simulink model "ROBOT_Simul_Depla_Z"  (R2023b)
settings: Solver=ode15s  StartTime=0.0  StopTime=0.2  RelTol=1e-3  EnableMultiTasking=on
undefined symbols (not defined in the file): BATI1_Défaut_sldprt, BATI2_Défaut_sldprt, BATI3_Défaut_sldprt, deg, kg, m, mm, N, rad, s, STL, X, Y, Z
libraries: sm_lib x139, fl_lib x42, nesl_utility x19, slpidlib x3
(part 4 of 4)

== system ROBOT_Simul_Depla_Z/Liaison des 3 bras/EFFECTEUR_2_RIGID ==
  ReferenceFrame : sm_lib/Frames and Transforms/Reference Frame
  Solid : sm_lib/Body Elements/File Solid  ExtGeomFileName=\STL\EFFECTEUR_Défaut_sldprt.STL  UnitType=Custom  ExtGeomFileUnits=mm  StepReaderType=HEX  ExportConvexHullGeometry=off  InertiaType=Custom  Mass=0.013453568991832839  MassUnits=kg  CenterOfMass=[-17.212650388480686 -9.9626588451280398 5.5774208666899616]  CenterOfMassUnits=mm  MomentsOfInertia=[1.2849612996466211 1.3154199043910564 2.2338709867359823]  MomentsOfInertiaUnits=kg*mm^2  ProductsOfInertia=[0.035925388048610812 0.056750034506765974 -0.058662844210309435]  ProductsOfInertiaUnits=kg*mm^2  BasedOnType=Density  Density=1000  DensityUnits=kg/(m^3)  DoExposeReferenceFrame=on  SerializedFrames=<Frames/>  GraphicType=FromGeometry  MarkerShape=Sphere  MarkerSize=10  MarkerSizeUnits=m  GraphicVisPropType=SimpleVisualProperties  GraphicDiffuseColor=[0.792156862745098 0.81960784313725488 0.93333333333333335]  GraphicSpecularColor=[0.5 0.5 0.5 1.0]  GraphicAmbientColor=[0.15 0.15 0.15 1.0]  GraphicEmissiveColor=[0.0 0.0 0.0 1.0]  GraphicShininess=75  GraphicOpacity=1
  F : PMIOPort  Side=Left
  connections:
  Solid/RConn1 -- ReferenceFrame/RConn1 -- F/RConn1

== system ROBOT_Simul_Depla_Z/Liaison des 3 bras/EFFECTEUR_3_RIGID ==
  ReferenceFrame : sm_lib/Frames and Transforms/Reference Frame
  Solid : sm_lib/Body Elements/File Solid  ExtGeomFileName=\STL\EFFECTEUR_Défaut_sldprt.STL  UnitType=Custom  ExtGeomFileUnits=mm  StepReaderType=HEX  ExportConvexHullGeometry=off  InertiaType=Custom  Mass=0.013453568991832839  MassUnits=kg  CenterOfMass=[-17.212650388480686 -9.9626588451280398 5.5774208666899616]  CenterOfMassUnits=mm  MomentsOfInertia=[1.2849612996466211 1.3154199043910564 2.2338709867359823]  MomentsOfInertiaUnits=kg*mm^2  ProductsOfInertia=[0.035925388048610812 0.056750034506765974 -0.058662844210309435]  ProductsOfInertiaUnits=kg*mm^2  BasedOnType=Density  Density=1000  DensityUnits=kg/(m^3)  DoExposeReferenceFrame=on  SerializedFrames=<Frames/>  GraphicType=FromGeometry  MarkerShape=Sphere  MarkerSize=10  MarkerSizeUnits=m  GraphicVisPropType=SimpleVisualProperties  GraphicDiffuseColor=[0.792156862745098 0.81960784313725488 0.93333333333333335]  GraphicSpecularColor=[0.5 0.5 0.5 1.0]  GraphicAmbientColor=[0.15 0.15 0.15 1.0]  GraphicEmissiveColor=[0.0 0.0 0.0 1.0]  GraphicShininess=75  GraphicOpacity=1
  F : PMIOPort  Side=Left
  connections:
  Solid/RConn1 -- ReferenceFrame/RConn1 -- F/RConn1

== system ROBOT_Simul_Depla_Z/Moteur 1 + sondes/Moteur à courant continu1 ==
  note: Kv = 1.18e-1
  Frottement : fl_lib/Mechanical/Rotational Elements/Rotational Friction  brkwy_trq=2.43e-3 N*m  brkwy_vel=0.030296 rad/s  Col_trq=2.43e-3 N*m  visc_coef=2e-6 N*m/(rad/s)  w_specify=off  w_priority=None  w=0 rad/s  w_nominal_specify=off  w_nominal_unit=rad/s  w_nominal_value=1  t_specify=off  t_priority=None  t=0 N*m  t_nominal_specify=off  t_nominal_unit=N*m  t_nominal_value=1
  Inductance induit 35mH : fl_lib/Electrical/Electrical Elements/Inductor  l=35 mH  r=0 Ohm  g=1e-09 1/Ohm  i_specify=off  i_priority=None  i=0 A  i_nominal_specify=off  i_nominal_unit=A  i_nominal_value=1  v_specify=off  v_priority=None  v=0 V  v_nominal_specify=off  v_nominal_unit=V  v_nominal_value=1  i_L_specify=on  i_L_priority=High  i_L=0 A  i_L_nominal_specify=off  i_L_nominal_unit=A  i_L_nominal_value=1
  Inertie Je 10e-6 : fl_lib/Mechanical/Rotational Elements/Inertia  inertia=10.5e-6 kg*m^2  num_ports=foundation.enum.numPorts2.one  w_specify=on  w_priority=High  w=0 rad/s  w_nominal_specify=off  w_nominal_unit=rad/s  w_nominal_value=1  t_specify=off  t_priority=None  t=0 N*m  t_nominal_specify=off  t_nominal_unit=N*m  t_nominal_value=1
  Moteur parfait : fl_lib/Electrical/Electrical Elements/Rotational Electromechanical Converter  K=1.18e-1 V/(rad/s)  i_specify=off  i_priority=None  i=0 A  i_nominal_specify=off  i_nominal_unit=A  i_nominal_value=1  v_specify=off  v_priority=None  v=0 V  v_nominal_specify=off  v_nominal_unit=V  v_nominal_value=1  t_specify=off  t_priority=None  t=0 N*m  t_nominal_specify=off  t_nominal_unit=N*m  t_nominal_value=1  w_specify=off  w_priority=None  w=0 rad/s  w_nominal_specify=off  w_nominal_unit=rad/s  w_nominal_value=1
  Rinduit 38 Ohms : fl_lib/Electrical/Electrical Elements/Resistor  Tag=Factory Generic  R=38 Ohm  i_specify=off  i_priority=None  i=0 A  i_nominal_specify=off  i_nominal_unit=A  i_nominal_value=1  v_specify=off  v_priority=None  v=0 V  v_nominal_specify=off  v_nominal_unit=V  v_nominal_value=1
  V+ : PMIOPort  Side=Left
  R : PMIOPort  Port=2  Side=Right
  C : PMIOPort  Port=3  Side=Right
  V- : PMIOPort  Port=4  Side=Left
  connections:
  C/RConn1 -- Moteur parfait/RConn2 -- Frottement/RConn1
  R/RConn1 -- Inertie Je 10e-6/LConn1 -- Moteur parfait/LConn2 -- Frottement/LConn1
  Inductance induit 35mH/LConn1 -- Rinduit 38 Ohms/RConn1
  Rinduit 38 Ohms/LConn1 -- V+/RConn1
  V-/RConn1 -- Moteur parfait/RConn1
  Moteur parfait/LConn1 -- Inductance induit 35mH/RConn1

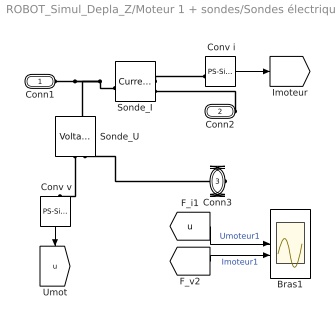
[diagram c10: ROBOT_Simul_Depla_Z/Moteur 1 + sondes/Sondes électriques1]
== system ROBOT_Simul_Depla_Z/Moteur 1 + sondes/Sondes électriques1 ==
  " Conv i" : nesl_utility/PS-Simulink Converter  PhysicalDomain=network_engine_domain  SubClassName=ps_output  LeftPortType=input  RightPortType=output  PseudoPeriodic=off  Frequencies=[]  VectorFormat=1-D array  Unit=1  AffineConversion=off
  " Conv v" : nesl_utility/PS-Simulink Converter  PhysicalDomain=network_engine_domain  SubClassName=ps_output  LeftPortType=input  RightPortType=output  PseudoPeriodic=off  Frequencies=[]  VectorFormat=1-D array  Unit=1  AffineConversion=off
  Bras1 : Scope  NumInputPorts=2
  Sonde_I : fl_lib/Electrical/Electrical Sensors/Current Sensor
  Sonde_U : fl_lib/Electrical/Electrical Sensors/Voltage Sensor
  Conn1 : PMIOPort  Side=Left
  Conn2 : PMIOPort  Port=2  Side=Right
  Conn3 : PMIOPort  Port=3  Side=Right
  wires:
  [i] -> Bras1/2  "Imoteur1"
  [u] -> Bras1/1  "Umoteur1"
  " Conv i"/1 -> [i]
  " Conv v"/1 -> [u]
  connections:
  Conn3/RConn1 -- Sonde_U/RConn2
  Conn2/RConn1 -- Sonde_I/RConn2
  Sonde_I/LConn1 -- Sonde_U/LConn1 -- Conn1/RConn1
  Sonde_U/RConn1 -- " Conv v"/LConn1
  Sonde_I/RConn1 -- " Conv i"/LConn1

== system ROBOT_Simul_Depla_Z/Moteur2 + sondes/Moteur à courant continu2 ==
  note: Kv = 1.18e-1
  Frottement : fl_lib/Mechanical/Rotational Elements/Rotational Friction  brkwy_trq=2.43e-3 N*m  brkwy_vel=0.030296 rad/s  Col_trq=2.43e-3 N*m  visc_coef=2e-6 N*m/(rad/s)  w_specify=off  w_priority=None  w=0 rad/s  w_nominal_specify=off  w_nominal_unit=rad/s  w_nominal_value=1  t_specify=off  t_priority=None  t=0 N*m  t_nominal_specify=off  t_nominal_unit=N*m  t_nominal_value=1
  Inductance induit 35mH : fl_lib/Electrical/Electrical Elements/Inductor  l=35 mH  r=0 Ohm  g=1e-09 1/Ohm  i_specify=off  i_priority=None  i=0 A  i_nominal_specify=off  i_nominal_unit=A  i_nominal_value=1  v_specify=off  v_priority=None  v=0 V  v_nominal_specify=off  v_nominal_unit=V  v_nominal_value=1  i_L_specify=on  i_L_priority=High  i_L=0 A  i_L_nominal_specify=off  i_L_nominal_unit=A  i_L_nominal_value=1
  Inertie Je 10e-6 : fl_lib/Mechanical/Rotational Elements/Inertia  inertia=10.5e-6 kg*m^2  num_ports=foundation.enum.numPorts2.one  w_specify=on  w_priority=High  w=0 rad/s  w_nominal_specify=off  w_nominal_unit=rad/s  w_nominal_value=1  t_specify=off  t_priority=None  t=0 N*m  t_nominal_specify=off  t_nominal_unit=N*m  t_nominal_value=1
  Moteur parfait : fl_lib/Electrical/Electrical Elements/Rotational Electromechanical Converter  K=1.18e-1 V/(rad/s)  i_specify=off  i_priority=None  i=0 A  i_nominal_specify=off  i_nominal_unit=A  i_nominal_value=1  v_specify=off  v_priority=None  v=0 V  v_nominal_specify=off  v_nominal_unit=V  v_nominal_value=1  t_specify=off  t_priority=None  t=0 N*m  t_nominal_specify=off  t_nominal_unit=N*m  t_nominal_value=1  w_specify=off  w_priority=None  w=0 rad/s  w_nominal_specify=off  w_nominal_unit=rad/s  w_nominal_value=1
  Rinduit 38 Ohms : fl_lib/Electrical/Electrical Elements/Resistor  Tag=Factory Generic  R=38 Ohm  i_specify=off  i_priority=None  i=0 A  i_nominal_specify=off  i_nominal_unit=A  i_nominal_value=1  v_specify=off  v_priority=None  v=0 V  v_nominal_specify=off  v_nominal_unit=V  v_nominal_value=1
  V+ : PMIOPort  Side=Left
  R : PMIOPort  Port=2  Side=Right
  C : PMIOPort  Port=3  Side=Right
  V- : PMIOPort  Port=4  Side=Left
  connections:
  Moteur parfait/LConn1 -- Inductance induit 35mH/RConn1
  V-/RConn1 -- Moteur parfait/RConn1
  Rinduit 38 Ohms/LConn1 -- V+/RConn1
  Inductance induit 35mH/LConn1 -- Rinduit 38 Ohms/RConn1
  Frottement/LConn1 -- Moteur parfait/LConn2 -- Inertie Je 10e-6/LConn1 -- R/RConn1
  Frottement/RConn1 -- Moteur parfait/RConn2 -- C/RConn1

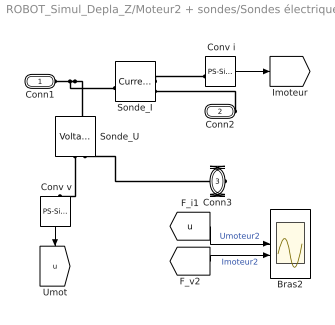
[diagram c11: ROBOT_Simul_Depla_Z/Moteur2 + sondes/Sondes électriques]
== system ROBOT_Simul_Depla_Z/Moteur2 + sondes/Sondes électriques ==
  " Conv i" : nesl_utility/PS-Simulink Converter  PhysicalDomain=network_engine_domain  SubClassName=ps_output  LeftPortType=input  RightPortType=output  PseudoPeriodic=off  Frequencies=[]  VectorFormat=1-D array  Unit=1  AffineConversion=off
  " Conv v" : nesl_utility/PS-Simulink Converter  PhysicalDomain=network_engine_domain  SubClassName=ps_output  LeftPortType=input  RightPortType=output  PseudoPeriodic=off  Frequencies=[]  VectorFormat=1-D array  Unit=1  AffineConversion=off
  Bras2 : Scope  NumInputPorts=2
  Sonde_I : fl_lib/Electrical/Electrical Sensors/Current Sensor
  Sonde_U : fl_lib/Electrical/Electrical Sensors/Voltage Sensor
  Conn1 : PMIOPort  Side=Left
  Conn2 : PMIOPort  Port=2  Side=Right
  Conn3 : PMIOPort  Port=3  Side=Right
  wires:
  " Conv v"/1 -> [u]
  " Conv i"/1 -> [i]
  [u] -> Bras2/1  "Umoteur2"
  [i] -> Bras2/2  "Imoteur2"
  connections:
  Sonde_I/RConn1 -- " Conv i"/LConn1
  Sonde_U/RConn1 -- " Conv v"/LConn1
  Conn1/RConn1 -- Sonde_U/LConn1 -- Sonde_I/LConn1
  Conn2/RConn1 -- Sonde_I/RConn2
  Conn3/RConn1 -- Sonde_U/RConn2

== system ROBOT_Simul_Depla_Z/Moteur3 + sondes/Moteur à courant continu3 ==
  note: Kv = 1.18e-1
  Frottement : fl_lib/Mechanical/Rotational Elements/Rotational Friction  brkwy_trq=2.43e-3 N*m  brkwy_vel=0.030296 rad/s  Col_trq=2.43e-3 N*m  visc_coef=2e-6 N*m/(rad/s)  w_specify=off  w_priority=None  w=0 rad/s  w_nominal_specify=off  w_nominal_unit=rad/s  w_nominal_value=1  t_specify=off  t_priority=None  t=0 N*m  t_nominal_specify=off  t_nominal_unit=N*m  t_nominal_value=1
  Inductance induit 35mH : fl_lib/Electrical/Electrical Elements/Inductor  l=35 mH  r=0 Ohm  g=1e-09 1/Ohm  i_specify=off  i_priority=None  i=0 A  i_nominal_specify=off  i_nominal_unit=A  i_nominal_value=1  v_specify=off  v_priority=None  v=0 V  v_nominal_specify=off  v_nominal_unit=V  v_nominal_value=1  i_L_specify=on  i_L_priority=High  i_L=0 A  i_L_nominal_specify=off  i_L_nominal_unit=A  i_L_nominal_value=1
  Inertie Je 10e-6 : fl_lib/Mechanical/Rotational Elements/Inertia  inertia=10.5e-6 kg*m^2  num_ports=foundation.enum.numPorts2.one  w_specify=on  w_priority=High  w=0 rad/s  w_nominal_specify=off  w_nominal_unit=rad/s  w_nominal_value=1  t_specify=off  t_priority=None  t=0 N*m  t_nominal_specify=off  t_nominal_unit=N*m  t_nominal_value=1
  Moteur parfait : fl_lib/Electrical/Electrical Elements/Rotational Electromechanical Converter  K=1.18e-1 V/(rad/s)  i_specify=off  i_priority=None  i=0 A  i_nominal_specify=off  i_nominal_unit=A  i_nominal_value=1  v_specify=off  v_priority=None  v=0 V  v_nominal_specify=off  v_nominal_unit=V  v_nominal_value=1  t_specify=off  t_priority=None  t=0 N*m  t_nominal_specify=off  t_nominal_unit=N*m  t_nominal_value=1  w_specify=off  w_priority=None  w=0 rad/s  w_nominal_specify=off  w_nominal_unit=rad/s  w_nominal_value=1
  Rinduit 38 Ohms : fl_lib/Electrical/Electrical Elements/Resistor  Tag=Factory Generic  R=38 Ohm  i_specify=off  i_priority=None  i=0 A  i_nominal_specify=off  i_nominal_unit=A  i_nominal_value=1  v_specify=off  v_priority=None  v=0 V  v_nominal_specify=off  v_nominal_unit=V  v_nominal_value=1
  V+ : PMIOPort  Side=Left
  R : PMIOPort  Port=2  Side=Right
  C : PMIOPort  Port=3  Side=Right
  V- : PMIOPort  Port=4  Side=Left
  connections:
  Moteur parfait/LConn1 -- Inductance induit 35mH/RConn1
  V-/RConn1 -- Moteur parfait/RConn1
  Rinduit 38 Ohms/LConn1 -- V+/RConn1
  Inductance induit 35mH/LConn1 -- Rinduit 38 Ohms/RConn1
  Frottement/LConn1 -- Moteur parfait/LConn2 -- Inertie Je 10e-6/LConn1 -- R/RConn1
  Frottement/RConn1 -- Moteur parfait/RConn2 -- C/RConn1

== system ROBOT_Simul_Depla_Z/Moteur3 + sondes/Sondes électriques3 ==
  " Conv i" : nesl_utility/PS-Simulink Converter  PhysicalDomain=network_engine_domain  SubClassName=ps_output  LeftPortType=input  RightPortType=output  PseudoPeriodic=off  Frequencies=[]  VectorFormat=1-D array  Unit=1  AffineConversion=off
  " Conv v" : nesl_utility/PS-Simulink Converter  PhysicalDomain=network_engine_domain  SubClassName=ps_output  LeftPortType=input  RightPortType=output  PseudoPeriodic=off  Frequencies=[]  VectorFormat=1-D array  Unit=1  AffineConversion=off
  Bras3 : Scope  NumInputPorts=2
  Sonde_I : fl_lib/Electrical/Electrical Sensors/Current Sensor
  Sonde_U : fl_lib/Electrical/Electrical Sensors/Voltage Sensor
  Conn1 : PMIOPort  Side=Left
  Conn2 : PMIOPort  Port=2  Side=Right
  Conn3 : PMIOPort  Port=3  Side=Right
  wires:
  " Conv v"/1 -> [u]
  " Conv i"/1 -> [i]
  [u] -> Bras3/1  "Umoteur3"
  [i] -> Bras3/2  "Imoteur3"
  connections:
  Sonde_I/RConn1 -- " Conv i"/LConn1
  Sonde_U/RConn1 -- " Conv v"/LConn1
  Conn1/RConn1 -- Sonde_U/LConn1 -- Sonde_I/LConn1
  Conn2/RConn1 -- Sonde_I/RConn2
  Conn3/RConn1 -- Sonde_U/RConn2

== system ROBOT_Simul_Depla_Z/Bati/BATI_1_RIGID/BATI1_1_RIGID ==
  ReferenceFrame : sm_lib/Frames and Transforms/Reference Frame
  Solid : sm_lib/Body Elements/File Solid  ExtGeomFileName=\STL\BATI1_Défaut_sldprt.STL  UnitType=Custom  ExtGeomFileUnits=mm  StepReaderType=HEX  ExportConvexHullGeometry=off  InertiaType=Custom  Mass=0.033663687372977959  MassUnits=kg  CenterOfMass=[20.336401330469712 25.63961437498785 5.3457144153831457]  CenterOfMassUnits=mm  MomentsOfInertia=[6.704545070550517 14.392527306394198 20.235421331927157]  MomentsOfInertiaUnits=kg*mm^2  ProductsOfInertia=[-0.10543470284856278 -0.074747369019470072 1.7068027580925555]  ProductsOfInertiaUnits=kg*mm^2  BasedOnType=Density  Density=1000  DensityUnits=kg/(m^3)  DoExposeReferenceFrame=on  SerializedFrames=<Frames/>  GraphicType=FromGeometry  MarkerShape=Sphere  MarkerSize=10  MarkerSizeUnits=m  GraphicVisPropType=SimpleVisualProperties  GraphicDiffuseColor=[0.75294117647058822 1 1]  GraphicSpecularColor=[0.5 0.5 0.5 1.0]  GraphicAmbientColor=[0.15 0.15 0.15 1.0]  GraphicEmissiveColor=[0.0 0.0 0.0 1.0]  GraphicShininess=75  GraphicOpacity=1
  F : PMIOPort  Side=Left
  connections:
  Solid/RConn1 -- ReferenceFrame/RConn1 -- F/RConn1

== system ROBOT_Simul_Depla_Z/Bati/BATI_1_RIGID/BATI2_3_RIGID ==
  ReferenceFrame : sm_lib/Frames and Transforms/Reference Frame
  Solid : sm_lib/Body Elements/File Solid  ExtGeomFileName=\STL\BATI2_Défaut_sldprt.STL  UnitType=Custom  ExtGeomFileUnits=mm  StepReaderType=HEX  ExportConvexHullGeometry=off  InertiaType=Custom  Mass=3.3661932429020234  MassUnits=kg  CenterOfMass=[20.336944533823793 25.639868756108907 5.3454769419575205]  CenterOfMassUnits=mm  MomentsOfInertia=[670.44550783613272 1439.2294811094996 2023.5171686685317]  MomentsOfInertiaUnits=kg*mm^2  ProductsOfInertia=[-10.547370497314642 -7.4830660580031543 170.68937998442982]  ProductsOfInertiaUnits=kg*mm^2  BasedOnType=Density  Density=1000  DensityUnits=kg/(m^3)  DoExposeReferenceFrame=on  SerializedFrames=<Frames/>  GraphicType=FromGeometry  MarkerShape=Sphere  MarkerSize=10  MarkerSizeUnits=m  GraphicVisPropType=SimpleVisualProperties  GraphicDiffuseColor=[0.75294117647058822 1 1]  GraphicSpecularColor=[0.5 0.5 0.5 1.0]  GraphicAmbientColor=[0.15 0.15 0.15 1.0]  GraphicEmissiveColor=[0.0 0.0 0.0 1.0]  GraphicShininess=75  GraphicOpacity=1
  F : PMIOPort  Side=Left
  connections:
  Solid/RConn1 -- ReferenceFrame/RConn1 -- F/RConn1

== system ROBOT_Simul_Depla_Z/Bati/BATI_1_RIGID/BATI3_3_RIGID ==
  ReferenceFrame : sm_lib/Frames and Transforms/Reference Frame
  Solid : sm_lib/Body Elements/File Solid  ExtGeomFileName=\STL\BATI3_Défaut_sldprt.STL  UnitType=Custom  ExtGeomFileUnits=mm  StepReaderType=HEX  ExportConvexHullGeometry=off  InertiaType=Custom  Mass=0.033661997544023686  MassUnits=kg  CenterOfMass=[20.336894016558855 25.639858086732207 5.3454859216357811]  CenterOfMassUnits=mm  MomentsOfInertia=[6.7044612586719987 14.392323903610993 20.235203785272009]  MomentsOfInertiaUnits=kg*mm^2  ProductsOfInertia=[-0.10547223942223864 -0.074822963165538006 1.706885098239038]  ProductsOfInertiaUnits=kg*mm^2  BasedOnType=Density  Density=1000  DensityUnits=kg/(m^3)  DoExposeReferenceFrame=on  SerializedFrames=<Frames/>  GraphicType=FromGeometry  MarkerShape=Sphere  MarkerSize=10  MarkerSizeUnits=m  GraphicVisPropType=SimpleVisualProperties  GraphicDiffuseColor=[0.75294117647058822 1 1]  GraphicSpecularColor=[0.5 0.5 0.5 1.0]  GraphicAmbientColor=[0.15 0.15 0.15 1.0]  GraphicEmissiveColor=[0.0 0.0 0.0 1.0]  GraphicShininess=75  GraphicOpacity=1
  F : PMIOPort  Side=Left
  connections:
  Solid/RConn1 -- ReferenceFrame/RConn1 -- F/RConn1

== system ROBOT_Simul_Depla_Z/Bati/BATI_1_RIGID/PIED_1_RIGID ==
  ReferenceFrame : sm_lib/Frames and Transforms/Reference Frame
  Solid : sm_lib/Body Elements/File Solid  ExtGeomFileName=\STL\PIED_Défaut_sldprt.STL  UnitType=Custom  ExtGeomFileUnits=mm  StepReaderType=HEX  ExportConvexHullGeometry=off  InertiaType=Custom  Mass=0.2400116994364806  MassUnits=kg  CenterOfMass=[-3.023797205330788 -10.775136940876026 -9.5034409989686353]  CenterOfMassUnits=mm  MomentsOfInertia=[1039.4350917464089 990.05262981218959 1785.3677193958695]  MomentsOfInertiaUnits=kg*mm^2  ProductsOfInertia=[91.936760537551947 25.766048207439965 -15.325521737410117]  ProductsOfInertiaUnits=kg*mm^2  BasedOnType=Density  Density=1000  DensityUnits=kg/(m^3)  DoExposeReferenceFrame=on  SerializedFrames=<Frames/>  GraphicType=FromGeometry  MarkerShape=Sphere  MarkerSize=10  MarkerSizeUnits=m  GraphicVisPropType=SimpleVisualProperties  GraphicDiffuseColor=[0.75294117647058822 1 1]  GraphicSpecularColor=[0.5 0.5 0.5 1.0]  GraphicAmbientColor=[0.15 0.15 0.15 1.0]  GraphicEmissiveColor=[0.0 0.0 0.0 1.0]  GraphicShininess=75  GraphicOpacity=1
  F : PMIOPort  Side=Left
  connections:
  Solid/RConn1 -- ReferenceFrame/RConn1 -- F/RConn1

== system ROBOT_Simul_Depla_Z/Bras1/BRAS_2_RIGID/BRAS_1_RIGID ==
  ReferenceFrame : sm_lib/Frames and Transforms/Reference Frame
  Solid : sm_lib/Body Elements/File Solid  ExtGeomFileName=\STL\BRAS_Défaut_sldprt.STL  UnitType=Custom  ExtGeomFileUnits=mm  StepReaderType=HEX  ExportConvexHullGeometry=off  InertiaType=Custom  Mass=0.044838950955509597  MassUnits=kg  CenterOfMass=[-9.0418534412108452e-05 8.4657112225167754 0.00015611796423892563]  CenterOfMassUnits=mm  MomentsOfInertia=[5.1909513043126365 1.33138621334256 4.0048796257842971]  MomentsOfInertiaUnits=kg*mm^2  ProductsOfInertia=[-7.521699658868721e-06 -1.2077060782263442e-05 -1.0591378087356949e-05]  ProductsOfInertiaUnits=kg*mm^2  BasedOnType=Density  Density=1000  DensityUnits=kg/(m^3)  DoExposeReferenceFrame=on  SerializedFrames=<Frames/>  GraphicType=FromGeometry  MarkerShape=Sphere  MarkerSize=10  MarkerSizeUnits=m  GraphicVisPropType=SimpleVisualProperties  GraphicDiffuseColor=[0.69803921568627447 0.69803921568627447 0.69803921568627447]  GraphicSpecularColor=[0.5 0.5 0.5 1.0]  GraphicAmbientColor=[0.15 0.15 0.15 1.0]  GraphicEmissiveColor=[0.0 0.0 0.0 1.0]  GraphicShininess=75  GraphicOpacity=1
  F : PMIOPort  Side=Left
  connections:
  Solid/RConn1 -- ReferenceFrame/RConn1 -- F/RConn1

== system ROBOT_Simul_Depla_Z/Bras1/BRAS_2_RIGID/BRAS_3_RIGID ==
  ReferenceFrame : sm_lib/Frames and Transforms/Reference Frame
  Solid : sm_lib/Body Elements/File Solid  ExtGeomFileName=\STL\BRAS_Défaut_sldprt.STL  UnitType=Custom  ExtGeomFileUnits=mm  StepReaderType=HEX  ExportConvexHullGeometry=off  InertiaType=Custom  Mass=0.044838950955509597  MassUnits=kg  CenterOfMass=[-9.0418534412108452e-05 8.4657112225167754 0.00015611796423892563]  CenterOfMassUnits=mm  MomentsOfInertia=[5.1909513043126365 1.33138621334256 4.0048796257842971]  MomentsOfInertiaUnits=kg*mm^2  ProductsOfInertia=[-7.521699658868721e-06 -1.2077060782263442e-05 -1.0591378087356949e-05]  ProductsOfInertiaUnits=kg*mm^2  BasedOnType=Density  Density=1000  DensityUnits=kg/(m^3)  DoExposeReferenceFrame=on  SerializedFrames=<Frames/>  GraphicType=FromGeometry  MarkerShape=Sphere  MarkerSize=10  MarkerSizeUnits=m  GraphicVisPropType=SimpleVisualProperties  GraphicDiffuseColor=[0.6 0.6 0.6]  GraphicSpecularColor=[0.5 0.5 0.5 1.0]  GraphicAmbientColor=[0.15 0.15 0.15 1.0]  GraphicEmissiveColor=[0.0 0.0 0.0 1.0]  GraphicShininess=75  GraphicOpacity=1
  F : PMIOPort  Side=Left
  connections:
  Solid/RConn1 -- ReferenceFrame/RConn1 -- F/RConn1

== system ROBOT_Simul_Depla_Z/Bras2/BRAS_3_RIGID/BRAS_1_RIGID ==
  ReferenceFrame : sm_lib/Frames and Transforms/Reference Frame
  Solid : sm_lib/Body Elements/File Solid  ExtGeomFileName=\STL\BRAS_Défaut_sldprt.STL  UnitType=Custom  ExtGeomFileUnits=mm  StepReaderType=HEX  ExportConvexHullGeometry=off  InertiaType=Custom  Mass=0.044838950955509597  MassUnits=kg  CenterOfMass=[-9.0418534412108452e-05 8.4657112225167754 0.00015611796423892563]  CenterOfMassUnits=mm  MomentsOfInertia=[5.1909513043126365 1.33138621334256 4.0048796257842971]  MomentsOfInertiaUnits=kg*mm^2  ProductsOfInertia=[-7.521699658868721e-06 -1.2077060782263442e-05 -1.0591378087356949e-05]  ProductsOfInertiaUnits=kg*mm^2  BasedOnType=Density  Density=1000  DensityUnits=kg/(m^3)  DoExposeReferenceFrame=on  SerializedFrames=<Frames/>  GraphicType=FromGeometry  MarkerShape=Sphere  MarkerSize=10  MarkerSizeUnits=m  GraphicVisPropType=SimpleVisualProperties  GraphicDiffuseColor=[0.69803921568627447 0.69803921568627447 0.69803921568627447]  GraphicSpecularColor=[0.5 0.5 0.5 1.0]  GraphicAmbientColor=[0.15 0.15 0.15 1.0]  GraphicEmissiveColor=[0.0 0.0 0.0 1.0]  GraphicShininess=75  GraphicOpacity=1
  F : PMIOPort  Side=Left
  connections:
  Solid/RConn1 -- ReferenceFrame/RConn1 -- F/RConn1

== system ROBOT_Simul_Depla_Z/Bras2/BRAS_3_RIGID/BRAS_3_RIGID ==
  ReferenceFrame : sm_lib/Frames and Transforms/Reference Frame
  Solid : sm_lib/Body Elements/File Solid  ExtGeomFileName=\STL\BRAS_Défaut_sldprt.STL  UnitType=Custom  ExtGeomFileUnits=mm  StepReaderType=HEX  ExportConvexHullGeometry=off  InertiaType=Custom  Mass=0.044838950955509597  MassUnits=kg  CenterOfMass=[-9.0418534412108452e-05 8.4657112225167754 0.00015611796423892563]  CenterOfMassUnits=mm  MomentsOfInertia=[5.1909513043126365 1.33138621334256 4.0048796257842971]  MomentsOfInertiaUnits=kg*mm^2  ProductsOfInertia=[-7.521699658868721e-06 -1.2077060782263442e-05 -1.0591378087356949e-05]  ProductsOfInertiaUnits=kg*mm^2  BasedOnType=Density  Density=1000  DensityUnits=kg/(m^3)  DoExposeReferenceFrame=on  SerializedFrames=<Frames/>  GraphicType=FromGeometry  MarkerShape=Sphere  MarkerSize=10  MarkerSizeUnits=m  GraphicVisPropType=SimpleVisualProperties  GraphicDiffuseColor=[0.6 0.6 0.6]  GraphicSpecularColor=[0.5 0.5 0.5 1.0]  GraphicAmbientColor=[0.15 0.15 0.15 1.0]  GraphicEmissiveColor=[0.0 0.0 0.0 1.0]  GraphicShininess=75  GraphicOpacity=1
  F : PMIOPort  Side=Left
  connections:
  Solid/RConn1 -- ReferenceFrame/RConn1 -- F/RConn1

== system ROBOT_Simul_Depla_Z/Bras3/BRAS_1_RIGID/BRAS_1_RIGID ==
  ReferenceFrame : sm_lib/Frames and Transforms/Reference Frame
  Solid : sm_lib/Body Elements/File Solid  ExtGeomFileName=\STL\BRAS_Défaut_sldprt.STL  UnitType=Custom  ExtGeomFileUnits=mm  StepReaderType=HEX  ExportConvexHullGeometry=off  InertiaType=Custom  Mass=0.044838950955509597  MassUnits=kg  CenterOfMass=[-9.0418534412108452e-05 8.4657112225167754 0.00015611796423892563]  CenterOfMassUnits=mm  MomentsOfInertia=[5.1909513043126365 1.33138621334256 4.0048796257842971]  MomentsOfInertiaUnits=kg*mm^2  ProductsOfInertia=[-7.521699658868721e-06 -1.2077060782263442e-05 -1.0591378087356949e-05]  ProductsOfInertiaUnits=kg*mm^2  BasedOnType=Density  Density=1000  DensityUnits=kg/(m^3)  DoExposeReferenceFrame=on  SerializedFrames=<Frames/>  GraphicType=FromGeometry  MarkerShape=Sphere  MarkerSize=10  MarkerSizeUnits=m  GraphicVisPropType=SimpleVisualProperties  GraphicDiffuseColor=[0.69803921568627447 0.69803921568627447 0.69803921568627447]  GraphicSpecularColor=[0.5 0.5 0.5 1.0]  GraphicAmbientColor=[0.15 0.15 0.15 1.0]  GraphicEmissiveColor=[0.0 0.0 0.0 1.0]  GraphicShininess=75  GraphicOpacity=1
  F : PMIOPort  Side=Left
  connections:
  Solid/RConn1 -- ReferenceFrame/RConn1 -- F/RConn1

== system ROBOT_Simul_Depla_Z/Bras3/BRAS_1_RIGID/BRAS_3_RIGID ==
  ReferenceFrame : sm_lib/Frames and Transforms/Reference Frame
  Solid : sm_lib/Body Elements/File Solid  ExtGeomFileName=\STL\BRAS_Défaut_sldprt.STL  UnitType=Custom  ExtGeomFileUnits=mm  StepReaderType=HEX  ExportConvexHullGeometry=off  InertiaType=Custom  Mass=0.044838950955509597  MassUnits=kg  CenterOfMass=[-9.0418534412108452e-05 8.4657112225167754 0.00015611796423892563]  CenterOfMassUnits=mm  MomentsOfInertia=[5.1909513043126365 1.33138621334256 4.0048796257842971]  MomentsOfInertiaUnits=kg*mm^2  ProductsOfInertia=[-7.521699658868721e-06 -1.2077060782263442e-05 -1.0591378087356949e-05]  ProductsOfInertiaUnits=kg*mm^2  BasedOnType=Density  Density=1000  DensityUnits=kg/(m^3)  DoExposeReferenceFrame=on  SerializedFrames=<Frames/>  GraphicType=FromGeometry  MarkerShape=Sphere  MarkerSize=10  MarkerSizeUnits=m  GraphicVisPropType=SimpleVisualProperties  GraphicDiffuseColor=[0.69803921568627447 0.69803921568627447 0.69803921568627447]  GraphicSpecularColor=[0.5 0.5 0.5 1.0]  GraphicAmbientColor=[0.15 0.15 0.15 1.0]  GraphicEmissiveColor=[0.0 0.0 0.0 1.0]  GraphicShininess=75  GraphicOpacity=1
  F : PMIOPort  Side=Left
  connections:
  Solid/RConn1 -- ReferenceFrame/RConn1 -- F/RConn1

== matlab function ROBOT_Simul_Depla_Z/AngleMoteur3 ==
function anglmot3  = fcn(x,y,z)
%#codegen
x = x/1000; y = y/1000; z = z/1000;
a = 0.06;
b = 0.1025;
c = 0.014;
d = 0.01125;
e = 0.01125;
f = 0.025 ;
r = 0.03723;
s = 0.02733;
phi1 = -0.252; %radians
pu1 = x*cos(phi1) + y*sin(phi1);
pv1 = -x*sin(phi1) + y*cos(phi1);
pw1 = z+0.082; 
theta11 = acos((s+pv1-f)/b);
equ10 = pu1-r+c;
equ11 = (pw1^2)+(equ10^2)+(a^2)+2*a*equ10-(d+e+b*sin(theta11))^2;
equ12 = (pw1^2)+(equ10^2)+(a^2)-2*a*equ10-(d+e+b*sin(theta11))^2;
equ13 = -4*a*pw1;
equ14 = (equ13^2)-4*equ11*equ12;
t1 = -(sqrt(equ14)+equ13)/(2*equ11);
anglmot3 = (atan(t1)*2+0.2073)*7.627;

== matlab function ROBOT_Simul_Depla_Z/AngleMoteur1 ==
function anglmot1  = fcn(x,y,z)
%#codegen
x = x/1000; y = y/1000; z = z/1000;
a = 0.06;
b = 0.1025;
c = 0.014;
d = 0.01125;
e = 0.01125;
f = 0.025 ;
r = 0.03723;
s = 0.02733;
phi1 = 1.842; %radians
pu1 = x*cos(phi1) + y*sin(phi1);
pv1 = -x*sin(phi1) + y*cos(phi1);
pw1 = z+0.082; 
theta11 = acos((s+pv1-f)/b);
equ10 = pu1-r+c;
equ11 = (pw1^2)+(equ10^2)+(a^2)+2*a*equ10-(d+e+b*sin(theta11))^2;
equ12 = (pw1^2)+(equ10^2)+(a^2)-2*a*equ10-(d+e+b*sin(theta11))^2;
equ13 = -4*a*pw1;
equ14 = (equ13^2)-4*equ11*equ12;
t1 = -(sqrt(equ14)+equ13)/(2*equ11);
anglmot1 = (atan(t1)*2+0.2073)*7.627;

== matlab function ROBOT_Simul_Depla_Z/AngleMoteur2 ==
function anglmot2 = fcn(x,y,z)
%#codegen
x = x/1000; y = y/1000; z = z/1000;
a = 0.06;
b = 0.1025;
c = 0.014;
d = 0.01125;
e = 0.01125;
f = 0.025 ;
r = 0.03723;
s = 0.02733;
phi1 = 3.937; %radians
pu1 = x*cos(phi1) + y*sin(phi1);
pv1 = -x*sin(phi1) + y*cos(phi1);
pw1 = z+0.082; 
theta11 = acos((s+pv1-f)/b);
equ10 = pu1-r+c;
equ11 = (pw1^2)+(equ10^2)+(a^2)+2*a*equ10-(d+e+b*sin(theta11))^2;
equ12 = (pw1^2)+(equ10^2)+(a^2)-2*a*equ10-(d+e+b*sin(theta11))^2;
equ13 = -4*a*pw1;
equ14 = (equ13^2)-4*equ11*equ12;
t1 = -(sqrt(equ14)+equ13)/(2*equ11);
anglmot2 = (atan(t1)*2+0.2073)*7.627;
